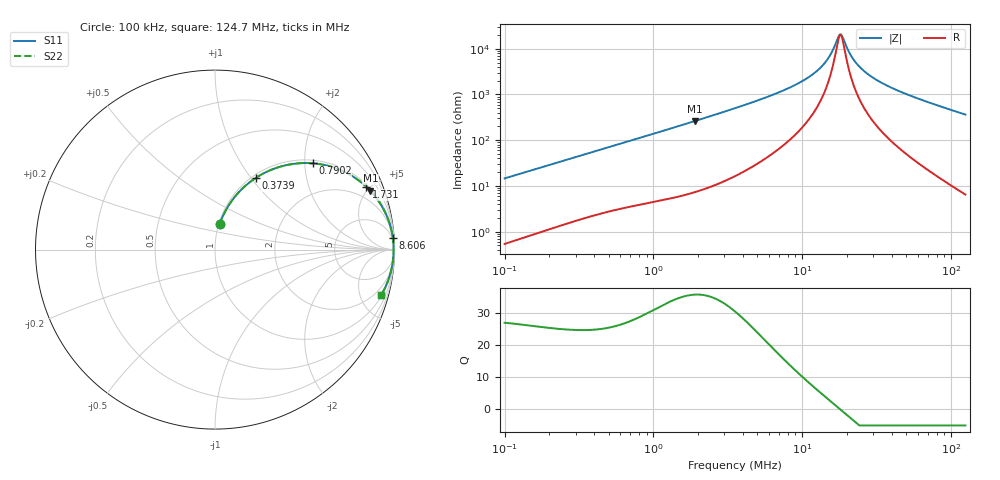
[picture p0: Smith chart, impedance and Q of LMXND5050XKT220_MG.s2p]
! LMXND5050XKT220_MG  S-PARAMETER MODEL  ( General Type )
! Model Generated by TAIYO YUDEN Corporation (http://www.ty-top.com)
! Version 1.0
! TAIYO YUDEN Control No. 191023NI43SB-FBB
! Copyright(c) 2019 TAIYO YUDEN CO.,LTD. All Rights Reserved.
! Product Description (link to TY-COMPAS)
! https://ds.yuden.co.jp/TYCOMPAS/or/detail?pn=LMXND5050XKT220MMG&u=M
! Products Name : Inductors
! Characteristics :
!  Inductance : 22 uH , SRF(min) : 13 MHz , DC Resistance(max) : 0.234 Ohm
!  Rated Current : Saturation :1400 mA , Temp Rise : 1050 mA
!  Case Size : 4.9 x 4.9 / 0.193 x 0.193 [mm/inch] , Thickness : 3 / 0.118 [mm/inch]
!  (Conditions: Temperature = 25 degC , DC Bias Current/Voltage = 0A / 0V)
! External Node Assignments :
!  1  o---GGG---o  2
! GND o---------o GND
! Frequency Range : 0.1MHz  -  124.6553MHz  [ 402 STEP ]
# MHz S RI R 50
! Freq[MHz].  S11 Real  S11 Imag  S21 Real  S21 Imag  S12 Real  S12 Imag  S22 Real  S22 Imag
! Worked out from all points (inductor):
!   401 points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, 100 kHz to 124.7 MHz, reference 50 ohm
!   read as one part in series: L = 23.1 uH near 103.6 kHz
!   highest Q = 35.9 at 1.892 MHz (marker M1), where L = 22 uH
!   self-resonance near 17.87 MHz
!   S11 on the Smith chart (normalised r, x): 100 kHz: 1.01, +0.29; 373.9 kHz: 1.04, +1.06; 790.2 kHz: 1.08, +2.19; 1.731 MHz: 1.13, +4.78; 8.606 MHz: 3, +30; 124.7 MHz: 1.13, -7.26
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0.1  0.0259 0.1413  0.9741 -0.1413  0.9741 -0.1413  0.0259 0.1413
0.193354  0.0803 0.2529  0.9197 -0.2529  0.9197 -0.2529  0.0803 0.2529
0.330013  0.1893 0.3721  0.8107 -0.3721  0.8107 -0.3721  0.1893 0.3721
0.373858  0.2272 0.3994  0.7728 -0.3994  0.7728 -0.3994  0.2272 0.3994
0.790235  0.5437 0.481  0.4563 -0.481  0.4563 -0.481  0.5437 0.481
1.089088  0.6876 0.4481  0.3124 -0.4481  0.3124 -0.4481  0.6876 0.4481
1.730949  0.8441 0.3491  0.1559 -0.3491  0.1559 -0.3491  0.8441 0.3491
1.892259  0.8656 0.3274  0.1344 -0.3274  0.1344 -0.3274  0.8656 0.3274
3.530656  0.9559 0.1897  0.0441 -0.1897  0.0441 -0.1897  0.9559 0.1897
8.606354  0.9907 0.0649  0.00929 -0.0649  0.00929 -0.0649  0.9907 0.0649
11.65164  0.9938 0.0363  0.00622 -0.0363  0.00622 -0.0363  0.9938 0.0363
14.42973  0.9948 0.0181  0.00517 -0.0181  0.00517 -0.0181  0.9948 0.0181
15.77446  0.9951 0.0108  0.00494 -0.0108  0.00494 -0.0108  0.9951 0.0108
17.55457  0.9952 0.00219  0.00481 -0.00219  0.00481 -0.00219  0.9952 0.00219
18.19151  0.9952 -0.00068  0.0048 0.00068  0.0048 0.00068  0.9952 -0.00068
18.85157  0.9952 -0.00355  0.00481 0.00355  0.00481 0.00355  0.9952 -0.00355
21.35612  0.995 -0.0137  0.00497 0.0137  0.00497 0.0137  0.995 -0.0137
24.19342  0.9946 -0.024  0.00536 0.024  0.00536 0.024  0.9946 -0.024
29.43265  0.9935 -0.041  0.00646 0.041  0.00646 0.041  0.9935 -0.041
38.45196  0.9907 -0.0667  0.00925 0.0667  0.00925 0.0667  0.9907 -0.0667
63.33127  0.9785 -0.1278  0.0215 0.1278  0.0215 0.1278  0.9785 -0.1278
124.6553  0.9257 -0.2536  0.0743 0.2536  0.0743 0.2536  0.9257 -0.2536
